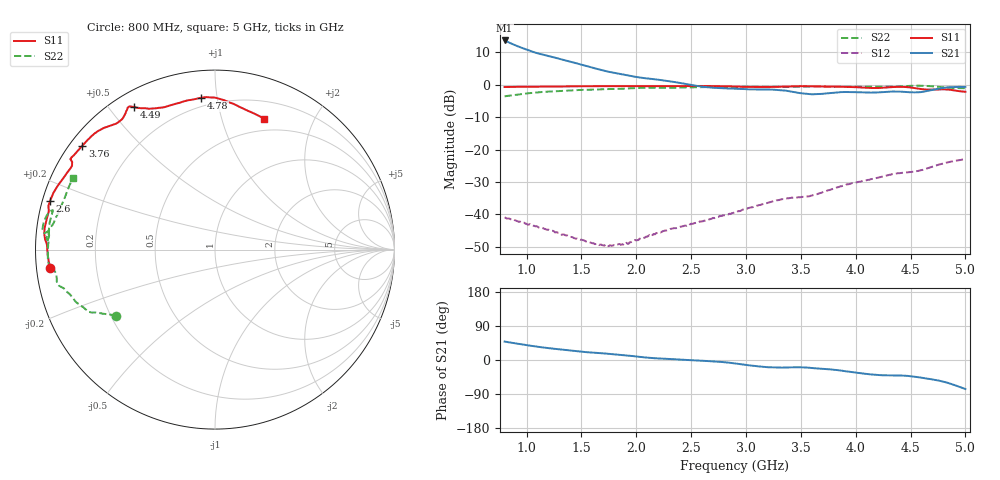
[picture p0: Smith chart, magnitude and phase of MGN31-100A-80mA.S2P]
! Port[1] = GATE
! Port[2] = DRAIN
! [Type]  S-parameter s2p file touchstone ver. 1.0
! [Object]  MGN31-100A
! [Bias]  80 mA
! [Version]  1.0
! [Date]  October, 2026
! [Source]  This file was created in JSC "ICC Milandr".
! [Disclaimer] Property of JSC "ICC Milandr". Unauthorized reproduction and/or distribution is strictly prohibited.
!  The file and the data are provided "AS IS" and with all faults and disclaim all warranties, express and implied, including
!  without limitation any implied warranties of merchantability, fitness for a particular purpose.
!  JSC "ICC Milandr" assumes no liability for:
!  1) the accuracy of the data provided;
!  2) the proper functioning of this data;
!  3) infringement of patents, copyrights or intellectual property rights resulting from the use of this data.
!  JSC "ICC Milandr" reserves the right to make changes to the products and the data without prior notice.
!  Please, be aware that your receipt and use of the file provided shall serve as acceptance of these terms and conditions.
!  If you do not accept these terms, you should return or destroy this file and any other accompanying information immediately.
# GHZ S MA R 50
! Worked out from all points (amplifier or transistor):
!   421 points, 800 MHz to 5 GHz, reference 50 ohm
!   highest |S21| = 13.7 dB at 800 MHz (marker M1)
!   |S21| within 3 dB of that: start of sweep to 1.014 GHz
!   unconditionally stable (mu >= 1): 1.43 GHz to 2.204 GHz; 2.218625 GHz to 2.223986 GHz
!   at 1.5 GHz: K = 1.07, MAG = 25.4 dB, |S12| = -47.8 dB
!   at 2.9 GHz: K = 0.59, MSG = 19.0 dB, |S12| = -39.3 dB
!   at 5 GHz: K = 0.39, MSG = 11.2 dB, |S12| = -23.0 dB
!   S11 on the Smith chart (normalised r, x): 800 MHz: 0.04, -0.05; 2.6 GHz: 0.02, +0.14; 3.76 GHz: 0.04, +0.35; 4.49 GHz: 0.06, +0.58; 4.78 GHz: 0.15, +0.90; 5 GHz: 0.37, +1.38
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0.8  0.923 -173.7  4.83 48.6  0.008991 -25.0  0.6611 -146.1
0.88  0.927 -175.4  4.194 44.7  0.008357 -26.7  0.6925 -148.6
0.94  0.9298 -176.7  3.818 41.9  0.007735 -27.2  0.7146 -149.9
1.02  0.9328 -178.5  3.389 38.3  0.006954 -27.9  0.7402 -151.5
1.09  0.9342 -179.9  3.098 35.5  0.006591 -28.5  0.7603 -152.6
1.25  0.938 178.0  2.645 29.8  0.005473 -26.3  0.7915 -154.9
1.5  0.9486 176.5  2.043 21.9  0.00408 -12.5  0.8324 -160.2
1.76  0.9563 174.0  1.572 16.1  0.003333 13.7  0.8598 -164.2
2  0.9524 169.2  1.318 9.3  0.003949 39.1  0.8901 -166.9
2.2  0.9523 166.5  1.196 4.2  0.005165 49.2  0.8963 -169.6
2.6  0.9582 163.6  0.9329 -2.0  0.007806 61.9  0.9214 -173.0
2.9  0.9389 156.1  0.8684 -9.1  0.01086 61.8  0.9288 -175.0
3.22  0.925 149.4  0.8421 -19.4  0.01545 57.7  0.9305 178.5
3.42  0.9462 148.0  0.7847 -19.2  0.01816 60.4  0.9298 174.4
3.6  0.9472 146.5  0.7137 -21.2  0.01946 60.4  0.9409 175.5
3.76  0.939 141.9  0.7422 -24.5  0.02367 58.3  0.9334 176.8
4.3  0.913 123.0  0.7803 -40.7  0.04035 42.0  0.9289 166.5
4.49  0.912 119.5  0.7667 -42.4  0.04475 39.2  0.9619 169.7
4.65  0.8416 108.5  0.7984 -49.0  0.05114 32.2  0.9595 174.3
4.78  0.8493 95.2  0.8843 -55.8  0.0599 25.2  0.9208 172.0
4.86  0.8377 87.5  0.9171 -62.1  0.06447 18.8  0.8973 167.1
5  0.7798 69.4  0.9272 -76.6  0.0711 4.9  0.8856 153.1
